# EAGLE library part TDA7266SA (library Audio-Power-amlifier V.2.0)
7W+7W DUAL BRIDGE AMPLIFIER
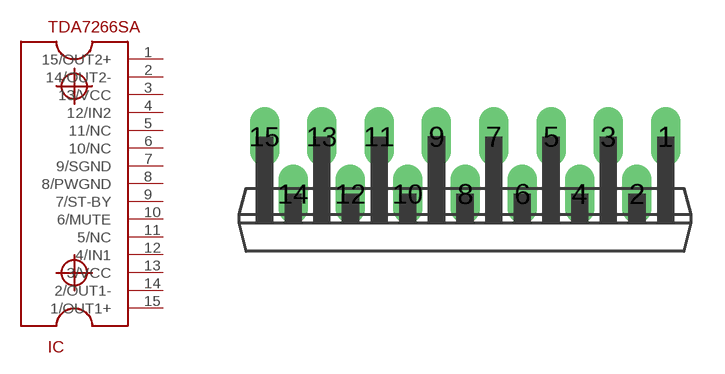
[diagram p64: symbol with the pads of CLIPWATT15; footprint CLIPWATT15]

Designator prefix IC

## TDA7266SA  [CLIPWATT15]
1  15/OUT2+  out
2  14/OUT2-  out
3  13/VCC  pwr
4  12/IN2  in
5  11/NC  nc
6  10/NC  nc
7  9/SGND  pwr
8  8/PWGND  pwr
9  7/ST-BY
10  6/MUTE
11  5/NC  nc
12  4/IN1  in
13  3/VCC  pwr
14  2/OUT1-  out
15  1/OUT1+  out

## Footprint CLIPWATT15 (pad centres in mm)
drill 0.8 pad 1.27 long: 1 8.89,2.54; 2 7.62,0; 3 6.35,2.54; 4 5.08,0; 5 3.81,2.54; 6 2.54,0; 7 1.27,2.54; 8 0,0; 9 -1.27,2.54; 10 -2.54,0; 11 -3.81,2.54; 12 -5.08,0; 13 -6.35,2.54; 14 -7.62,0; 15 -8.89,2.54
